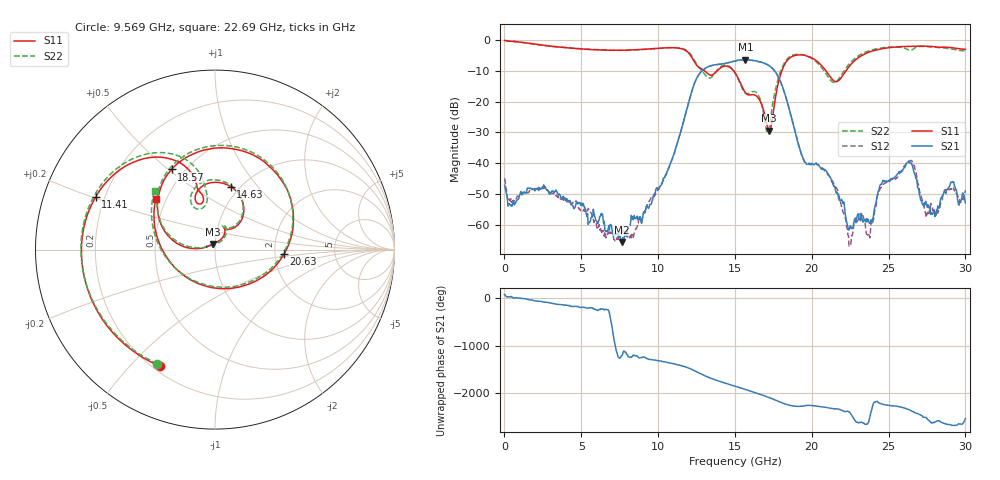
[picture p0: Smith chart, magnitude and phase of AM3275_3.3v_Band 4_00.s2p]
!Keysight Technologies,N5245B,MY58422270,A.16.20.02
!Date: Thursday, March 27, 2025 02:05:09
!Correction: S11(C  2-Port  )
!S21(C  2-Port  )
!S12(C  2-Port  )
!S22(C  2-Port  )
!S2P File: Measurements: S11, S21, S12, S22:
# Hz S  dB  R 50
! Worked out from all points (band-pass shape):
!   801 points, 10 MHz to 30 GHz, reference 50 ohm
!   highest |S21| = -6.45 dB at 15.68 GHz (marker M1); lowest = -65.5 dB at 7.62 GHz (marker M2)
!   |S21| within 3 dB of the highest: 13.01 GHz to 17.48 GHz (4.468 GHz wide, 29.3 % of centre)
!   lowest |S11| = -29.4 dB at 17.22 GHz (marker M3), VSWR 1.07, Z = 48.7 + j3.08 ohm
!   |S11| at or under -10 dB: 13.01 GHz to 13.85 GHz (845.4 MHz wide, 6.29 % of centre); 14.91 GHz to 18.05 GHz (3.146 GHz wide, 19.1 % of centre); 20.92 GHz to 22.23 GHz (1.31 GHz wide, 6.07 % of centre)
!   |S22| runs from -29.9 to -0.2 dB; largest |S21 - S12| = 0.0083
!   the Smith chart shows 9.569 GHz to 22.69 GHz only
!   S11 on the Smith chart (normalised r, x): 9.569 GHz: 0.23, -0.61; 11.41 GHz: 0.17, +0.21; 14.63 GHz: 0.91, +0.73; 18.57 GHz: 0.43, +0.51; 20.63 GHz: 2.25, -0.13; 22.69 GHz: 0.44, +0.31
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1e7  -0.22 -3.9  -47.03 71.4  -44.81 160.8  -0.22 -4.9
1.172112e9  -0.85 -83.0  -50.10 -12.5  -49.45 -13.0  -0.88 -83.1
2.521662e9  -1.79 -161.4  -47.66 -83.8  -48.11 -85.1  -1.77 -161.6
5.033325e9  -2.98 85.5  -52.86 165.4  -55.58 165.5  -2.89 84.7
7.619962e9  -3.39 -25.4  -65.46 -133.1  -62.25 -68.3  -3.41 -27.2
9.569312e9  -2.89 -115.2  -53.04 146.8  -50.87 149.7  -2.95 -116.8
1.001916e10  -2.73 -136.0  -48.51 124.4  -48.31 121.7  -2.78 -137.5
1.14062e10  -2.77 156.2  -30.85 28.2  -30.90 28.0  -2.66 155.5
1.305565e10  -10.19 102.9  -9.29 164.3  -9.29 164.2  -11.31 99.5
1.463012e10  -8.83 76.0  -7.34 -13.9  -7.35 -13.8  -8.60 77.2
1.5005e10  -10.66 57.3  -6.84 -51.1  -6.84 -51.1  -10.64 57.8
1.567978e10  -17.08 54.2  -6.45 -120.8  -6.45 -120.9  -17.29 61.3
1.721676e10  -29.45 110.6  -8.36 70.8  -8.36 70.8  -28.80 140.0
1.856631e10  -5.89 118.5  -22.98 -92.9  -23.01 -93.5  -5.49 115.0
2.002832e10  -5.92 33.4  -40.06 -99.9  -40.19 -99.2  -6.16 29.3
2.062812e10  -8.27 -3.6  -41.87 -124.1  -41.19 -120.6  -8.93 -9.6
2.268994e10  -7.23 139.2  -60.76 8.7  -61.51 -98.6  -6.54 135.7
2.37021e10  -4.04 92.6  -58.56 -80.3  -62.57 -95.1  -3.63 91.3
2.501416e10  -2.58 50.8  -45.48 -94.7  -45.57 -97.3  -2.36 48.7
2.651366e10  -2.11 10.1  -40.24 144.4  -39.14 138.5  -3.30 13.1
2.748834e10  -2.10 -17.4  -53.47 -5.1  -56.17 -77.8  -2.19 -17.1
3e10  -3.09 -108.6  -52.80 -11.4  -48.69 -132.5  -3.52 -108.7
